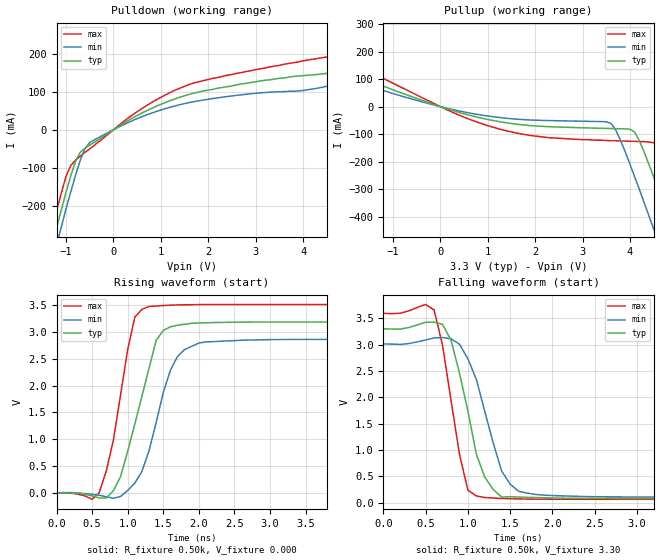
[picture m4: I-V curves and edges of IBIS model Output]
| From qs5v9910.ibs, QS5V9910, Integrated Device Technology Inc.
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|   Model Output
[Model]   Output
Model_type   Output
Polarity   Inverting
Vmeas =  1.500V
C_comp   5.00pF   5.00pF   5.00pF
[Temperature Range]   25.00   85.00   -40.00
[Voltage Range]   3.30V   3.00V   3.60V
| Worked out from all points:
|   slope of the pulldown table from 0 to 0.495 V, typ, clamps not added: 13.4 ohm
|   slope of the pullup table from 0 to 0.495 V, typ, clamps not added: 19.1 ohm
|   rising waveform, R_fixture 0.50k, V_fixture 0.000: 20-80 % time 373ps typ, 358ps min, 272ps max; typ from 0 V to 3.19 V
|   falling waveform, R_fixture 0.50k, V_fixture 3.30: 20-80 % time 276ps typ, 307ps min, 213ps max; typ from 3.3 V to 0.079 V
[Pulldown]
| voltage   I(typ)   I(min)   I(max)
-3.3V     -1.281A    -1.326A    -1.232A
-1.5V     -398mA     -445mA     -348mA
-1V       -164mA     -208mA     -122mA
-800mV    -83.04mA   -120mA     -79.75mA
-600mV    -48.54mA   -49.28mA   -59.59mA
-500mV    -40.52mA   -33.64mA   -50.12mA
500mV     37.32mA    29.14mA    47.42mA
1.3V      81.04mA    62.59mA    104mA
2.1V      106mA      81.91mA    135mA
4.9V      159mA      127mA      200mA
6.1V      215mA      176mA      263mA
6.6V      244mA      201mA      299mA
[Pullup]
| voltage   I(typ)   I(min)   I(max)
-3.3V     215mA      173mA      287mA
-800mV    48.44mA    37.33mA    67.98mA
800mV     -39.23mA   -28.78mA   -57.64mA
1.9V      -68.95mA   -48.58mA   -105mA
3.6V      -79.64mA   -61.02mA   -124mA
3.8V      -80.49mA   -123mA     -125mA
4.1V      -93.25mA   -256mA     -126mA
4.5V      -256mA     -445mA     -131mA
4.7V      -351mA     -542mA     -170mA
4.9V      -447mA     -639mA     -256mA
5.3V      -641mA     -835mA     -446mA
6.6V      -1.281A    -1.475A    -1.084A
[Ramp]
| variable   typ   min   max
dV/dt_r   1.91/0.37n   1.72/0.36n   2.11/0.27n
dV/dt_f   1.93/0.28n   1.75/0.31n   2.12/0.21n
R_load = 0.50k
[Rising Waveform]
R_fixture = 0.50k
V_fixture = 0.000
| time   V(typ)   V(min)   V(max)
0s        0V         0V         0V
600ps     -96.6mV    -44.88mV   1.523mV
800ps     38.69mV    -102mV     986mV
900ps     301mV      -68.17mV   1.827V
1.1ns     1.282V     180mV      3.277V
1.3ns     2.321V     785mV      3.478V
1.4ns     2.841V     1.309V     3.485V
1.6ns     3.097V     2.284V     3.502V
2ns       3.17V      2.794V     3.512V
9.9ns     3.187V     2.864V     3.514V
[Falling Waveform]
R_fixture = 0.50k
V_fixture = 3.30
| time   V(typ)   V(min)   V(max)
0s        3.3V       3.013V     3.593V
600ps     3.426V     3.127V     3.657V
700ps     3.384V     3.133V     2.989V
800ps     3.084V     3.112V     1.944V
900ps     2.463V     3.008V     922mV
1ns       1.74V      2.73V      235mV
1.1ns     918mV      2.341V     126mV
1.4ns     105mV      598mV      78.77mV
1.8ns     96.09mV    155mV      66.18mV
9.9ns     78.8mV     100mV      62.29mV
